| IBIS file generated by GenIBIS.exe Version 2.20
|   am37xxcbp
[IBIS ver]   4.1
[File name]   sprm509.ibs
[File Rev]   1.0
[Date]   Fri June 4, 2010, 5:00:0
[Source]   Data created at Texas Instruments
[Notes]   1) IBIS spec conformance checker (IBISCK4) ran with 0 errors
   and 576 warnings.  Warnings should be waived.
[Disclaimer] Please be aware that in the absence of a written agreement,
   Texas Instruments (TI) assumes no liability for: 1) the
   accuracy of the IBIS models provided to your company, 2) the
   proper functioning of these IBIS models in your design or for
   any resulting applications, or, 3) infringement of patents,
   copyrights, or intellectual property rights resulting from
   your use of these IBIS models. TI provides IBIS models as a
   service to our customers and therefore reserves the right to
   limit distribution of the IBIS models.
[Copyright]   Property of Texas Instruments Incorporated. Unauthorised
   reproduction and/or distribution is strictly prohibited. This
   product is protected under copyright law and trade secret law
   as an unpublished work. Created 1999,(C) Copyright 1999-2001,
   Texas Instruments Incorporated., All Rights Reserved. These
   commodities are under the U.S. Government distribution license
   control.As such,they are not to be re-exported without the
   prior approval of the U.S. Department of Commerce.
|   Component am37xxcbp
[Component]   am37xxcbp
[Manufacturer]   Texas Instruments.
[Package Model] am37xxcbp
[Package]
|   typ   min   max
R_pkg   0.39276334   6.43680e-004   7.84883e-001
L_pkg   4.201879E-009   -9.18420e-011   8.49560e-009
C_pkg   6.560845E-011   -1.66561e-011   1.47873e-010
[Pin]   signal_name   model_name
C27   CAM_PCLK   Selector2
C24   CAM_D3   Selector16
C23   CAM_FLD   Selector10
AH17   CAM_D1   Selector3
B26   CAM_XCLKB   Selector2
B25   CAM_D10   Selector8
A25   CAM_D5   Selector16
A24   CAM_HS   Selector10
K27   CAM_D8   Selector12
C26   CAM_D11   Selector8
D24   CAM_D4   Selector16
K28   CAM_D6   Selector12
L27   CAM_D9   Selector12
B24   CAM_D2   Selector16
L28   CAM_D7   Selector12
AG17   CAM_D0   Selector3
B23   CAM_WEN   Selector10
A23   CAM_VS   Selector10
C25   CAM_XCLKA   Selector2
D25   CAM_STROBE   Selector2
AG19   gpio_112   Selector12
AH19   gpio_113   Selector12
AG18   gpio_114   Selector12
AH18   gpio_115   Selector12
AD27   DSS_DATA11   Selector16
E27   DSS_ACBIAS   Selector8
D27   DSS_VSYNC   Selector8
H25   DSS_DATA19   Selector8
E28   DSS_DATA20   Selector8
AH23   DSS_DATA3   Selector15
H27   DSS_DATA17   Selector8
AB27   DSS_DATA13   Selector16
AC27   DSS_DATA22   Selector16
AG23   DSS_DATA2   Selector15
AD28   DSS_DATA10   Selector16
G26   DSS_DATA9   Selector8
AA27   DSS_DATA15   Selector16
AH24   DSS_DATA5   Selector15
D26   DSS_HSYNC   Selector8
AG22   DSS_DATA0   Selector13
AG24   DSS_DATA4   Selector15
H26   DSS_DATA18   Selector8
AB28   DSS_DATA12   Selector16
AH22   DSS_DATA1   Selector13
F28   DSS_DATA7   Selector8
AA28   DSS_DATA14   Selector16
G25   DSS_DATA16   Selector8
D28   DSS_PCLK   Selector8
J26   DSS_DATA21   Selector8
E26   DSS_DATA6   Selector8
AC28   DSS_DATA23   Selector16
F27   DSS_DATA8   Selector8
AE10   ETK_CTL   Selector2
AH12   ETK_D2   Selector2
AG7   ETK_D12   Selector2
AG8   ETK_D14   Selector2
AE11   ETK_D4   Selector2
AH8   ETK_D15   Selector2
AE7   ETK_D10   Selector2
AH7   ETK_D13   Selector2
AF11   ETK_D0   Selector2
AF10   ETK_CLK   Selector2
AG9   ETK_D9   Selector2
AG12   ETK_D1   Selector2
AE13   ETK_D3   Selector2
AH14   ETK_D7   Selector2
AF9   ETK_D8   Selector2
AF7   ETK_D11   Selector2
AH9   ETK_D5   Selector2
AF13   ETK_D6   Selector2
K8   GPMC_WAIT2   Selector16
T2   GPMC_D13   Selector8
U8   GPMC_NCS3   Selector16
M3   GPMC_A8   Selector16
V2   GPMC_D6   Selector8
H2   GPMC_D8   Selector8
L4   GPMC_A3   Selector8
H1   GPMC_NWP   Selector8
R8   GPMC_NCS5   Selector16
G3   GPMC_NBE0_CLE   Selector8
L3   GPMC_A9   Selector16
P8   GPMC_NCS6   Selector16
R3   GPMC_A6   Selector16
Y1   GPMC_D15   Selector8
H3   GPMC_NCS1   Selector16
T1   GPMC_D4   Selector8
K3   GPMC_A10   Selector16
L8   GPMC_WAIT1   Selector16
K1   GPMC_D0   Selector8
F3   GPMC_NADV_ALE   Selector16
V1   GPMC_D5   Selector8
R1   GPMC_D11   Selector8
T8   GPMC_NCS4   Selector16
L1   GPMC_D1   Selector8
G2   GPMC_NOE   Selector16
W2   GPMC_D7   Selector8
J8   GPMC_WAIT3   Selector16
M4   GPMC_A2   Selector8
P2   GPMC_D3   Selector8
K2   GPMC_D9   Selector8
W1   GPMC_D14   Selector8
K4   GPMC_A4   Selector8
G4   GPMC_NCS0   Selector16
M8   GPMC_WAIT0   Selector16
N3   GPMC_A7   Selector16
R2   GPMC_D12   Selector8
F4   GPMC_NWE   Selector16
U3   GPMC_NBE1   Selector8
N4   GPMC_A1   Selector8
V8   GPMC_NCS2   Selector16
T4   GPMC_CLK   Selector8
L2   GPMC_D2   Selector8
N8   GPMC_NCS7   Selector16
P1   GPMC_D10   Selector8
T3   GPMC_A5   Selector8
J25   HDQ_SIO   Selector5
U26   HSUSB0_DATA3   Selector2
R28   HSUSB0_DIR   Selector2
T27   HSUSB0_DATA0   Selector2
U27   HSUSB0_DATA2   Selector2
V28   HSUSB0_DATA5   Selector2
T25   HSUSB0_STP   Selector2
T26   HSUSB0_NXT   Selector2
U28   HSUSB0_DATA1   Selector2
U25   HSUSB0_DATA4   Selector2
V26   HSUSB0_DATA7   Selector2
T28   HSUSB0_CLK   Selector19
V27   HSUSB0_DATA6   Selector2
AF15   I2C2_SCL   Selector17
AG14   I2C3_SDA   Selector17
AD26   I2C4_SCL   Selector20
AF14   I2C3_SCL   Selector17
AE26   I2C4_SDA   Selector20
J21   I2C1_SDA   Selector17
AE15   I2C2_SDA   Selector17
K21   I2C1_SCL   Selector17
AA20   JTAG_TDI   Selector1
AA11   JTAG_EMU0   Selector1
AA12   JTAG_RTCK   Selector1
AA19   JTAG_TDO   Selector1
AA10   JTAG_EMU1   Selector1
AA13   JTAG_TCK   Selector1
AA18   JTAG_TMS_TMSC   Selector1
AA17   JTAG_NTRST   Selector1
T21   MCBSP_CLKS   Selector2
K26   MCBSP1_FSX   Selector2
W21   MCBSP1_CLKX   Selector2
AA21   MCBSP1_FSR   Selector2
V21   MCBSP1_DX   Selector2
Y21   MCBSP1_CLKR   Selector2
U21   MCBSP1_DR   Selector2
N21   MCBSP2_CLKX   Selector2
P21   MCBSP2_FSX   Selector2
R21   MCBSP2_DR   Selector2
M21   MCBSP2_DX   Selector2
AE5   MCBSP3_FSX   Selector2
AF5   MCBSP3_CLKX   Selector2
AF6   MCBSP3_DX   Selector2
AE6   MCBSP3_DR   Selector2
AD1   MCBSP4_DR   Selector2
AE1   MCBSP4_CLKX   Selector2
AD2   MCBSP4_DX   Selector2
AC1   MCBSP4_FSX   Selector2
AB1   MCSPI1_CS2   Selector2
AB2   MCSPI1_CS3   Selector2
AB4   MCSPI1_SIMO   Selector2
AC3   MCSPI1_CS1   Selector2
AA4   MCSPI1_SOMI   Selector2
AB3   MCSPI1_CLK   Selector2
AC2   MCSPI1_CS0   Selector2
AA3   MCSPI2_CLK   Selector2
V3   MCSPI2_CS1   Selector2
Y4   MCSPI2_CS0   Selector2
Y3   MCSPI2_SOMI   Selector2
Y2   MCSPI2_SIMO   Selector2
M27   MMC1_CMD   Selector14
N25   MMC1_DAT2   Selector14
N28   MMC1_CLK   Selector14
N27   MMC1_DAT0   Selector14
N26   MMC1_DAT1   Selector14
P28   MMC1_DAT3   Selector14
AE4   MMC2_DAT4   Selector2
AH4   MMC2_DAT1   Selector2
AG5   MMC2_CMD   Selector2
AH5   MMC2_DAT0   Selector2
AF3   MMC2_DAT6   Selector2
AF4   MMC2_DAT3   Selector2
AE2   MMC2_CLK   Selector2
AG4   MMC2_DAT2   Selector2
AE3   MMC2_DAT7   Selector2
AH3   MMC2_DAT5   Selector2
R27   gpio_128   Selector4
R25   gpio_129   Selector6
P27   gpio_126   Selector6
P26   gpio_127   Selector6
AF25   SYS_CLKREQ   Selector7
AG26   SYS_BOOT1   Selector8
AF18   SYS_BOOT3   Selector8
AH25   SYS_NRESPWRON   Model225
AE25   SYS_32K   Selector7
AF26   SYS_NIRQ   Selector18
AE21   SYS_BOOT5   Selector8
AF24   SYS_NRESWARM   Selector9
AE17   SYS_XTALIN   Model1
AG25   SYS_CLKOUT1   Selector11
AE14   SYS_BOOT2   Selector8
AF21   SYS_BOOT6   Selector16
AF19   SYS_BOOT4   Selector8
AH26   SYS_BOOT0   Selector8
AF22   SYS_OFF_MODE   Selector11
AE22   SYS_CLKOUT2   Selector10
Y8   UART1_RTS   Selector2
AA9   UART1_RX   Selector2
AA8   UART1_TX   Selector2
W8   UART1_CTS   Selector2
AB25   UART2_RTS   Selector10
AB26   UART2_CTS   Selector10
AA25   UART2_TX   Selector10
AD25   UART2_RX   Selector10
H20   UART3_RX_IRRX   Selector5
H21   UART3_TX_IRTX   Selector21
H18   UART3_CTS_RCTX   Selector5
H19   UART3_RTS_SD   Selector21
| Device pads which are not required to be modeled. Included for completeness
|U4   CAP_VDD_BB_MPU_IVA   POWER
|AH20   CAP_VDDU_ARRAY   POWER
|L21   CAP_VDD_SRAM_CORE   POWER
|AA15   CAP_VDDU_WKUP_LOGIC  POWER
|V4   CAP_VDD_SRAM_MPU_IVA POWER
|Y17   SYS_XTALGND   KELVINGROUND
|AC4   VDD_CORE   POWER
|AE18   VDD_CORE   POWER
|AE19   VDD_CORE   POWER
|AE24   VDD_CORE   POWER
|AE9   VDD_CORE   POWER
|D15   VDD_CORE   POWER
|D22   VDD_CORE   POWER
|D23   VDD_CORE   POWER
|D8   VDD_CORE   POWER
|D9   VDD_CORE   POWER
|E25   VDD_CORE   POWER
|H4   VDD_CORE   POWER
|J18   VDD_CORE   POWER
|J19   VDD_CORE   POWER
|J20   VDD_CORE   POWER
|J4   VDD_CORE   POWER
|K18   VDD_CORE   POWER
|K20   VDD_CORE   POWER
|L25   VDD_CORE   POWER
|M19   VDD_CORE   POWER
|M25   VDD_CORE   POWER
|N19   VDD_CORE   POWER
|N20   VDD_CORE   POWER
|P20   VDD_CORE   POWER
|T19   VDD_CORE   POWER
|U19   VDD_CORE   POWER
|U20   VDD_CORE   POWER
|V20   VDD_CORE   POWER
|W18   VDD_CORE   POWER
|W20   VDD_CORE   POWER
|Y16   VDD_CORE   POWER
|Y18   VDD_CORE   POWER
|Y19   VDD_CORE   POWER
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[Model Selector] Selector1
Model2 1.8V-I/O-PD-X-1.8V +5/-10%
Model3 1.8V-I/O-PI-X-1.8V +5/-10%V
Model4 1.8V-I/O-PU-X-1.8V +5/-10%
|   Usage I#1.8V#PD/PI/PU#LB0/LB1#BQ1850OMAPSMART2HYFBPB_SSBHH
[Model Selector] Selector2
Model10 1.8V-I/O-PI-LB1-1.8 +5/-10%
Model5 1.8V-I/O-PI-LB0-1.8 +5/-10%
Model6 1.8V-I/O-PU-LB0-1.8 +5/-10%
Model7 1.8V-I/O-PD-LB0-1.8 +5/-10%
Model8 1.8V-I/O-PU-LB1-1.8 +5/-10%
Model9 1.8V-I/O-PD-LB1-1.8 +5/-10%
|   Usage I#1.8V#PD/PI/PU##CAMERARX_ADDON.DY3
[Model Selector] Selector3
Model11 1.8V-INPUT-PD-X-1.8V +5/-10%
Model12 1.8V-INPUT-PI-X-1.8V +5/-10%
Model13 1.8V-INPUT-PU-X-1.8V +5/-10%
|   Usage O#1.8V#PD/PI/PU#SC00LB00/SC00LB01/SC01LB10/SC01LB11/SC10LB10/SC10LB11#BQ18OMAPSMART1HYFBPBNOPM_SSBHH
[Model Selector] Selector4
Model14 1.8V-I/O-PI-SC00LB00-1.8 +5/-10%
Model15 1.8V-I/O-PU-SC00LB00-1.8 +5/-10%
Model16 1.8V-I/O-PD-SC00LB00-1.8 +5/-10%
Model17 1.8V-I/O-PU-SC00LB01-1.8 +5/-10%
Model18 1.8V-I/O-PD-SC00LB01-1.8 +5/-10%
Model19 1.8V-I/O-PI-SC00LB01-1.8 +5/-10%
Model20 1.8V-I/O-PD-SC01LB10-1.8 +5/-10%
Model21 1.8V-I/O-PI-SC01LB10-1.8 +5/-10%
Model22 1.8V-I/O-PU-SC01LB10-1.8 +5/-10%
Model23 1.8V-I/O-PD-SC01LB11-1.8 +5/-10%
Model24 1.8V-I/O-PU-SC01LB11-1.8 +5/-10%
Model25 1.8V-I/O-PI-SC01LB11-1.8 +5/-10%
Model26 1.8V-I/O-PI-SC10LB10-1.8 +5/-10%
Model27 1.8V-I/O-PU-SC10LB10-1.8 +5/-10%
Model28 1.8V-I/O-PD-SC10LB10-1.8 +5/-10%
Model29 1.8V-I/O-PU-SC10LB11-1.8 +5/-10%
Model30 1.8V-I/O-PI-SC10LB11-1.8 +5/-10%
Model31 1.8V-I/O-PD-SC10LB11-1.8 +5/-10%
|   Usage I#1.8V#PD/PI/PU#SC00LB00/SC00LB01/SC01LB10/SC01LB11/SC10LB10/SC10LB11#BQ18OMAPSMART1HYFBPB_SSBHH
[Model Selector] Selector5
Model32 1.8V-I/O-PD-SC01LB11-1.8 +5/-10%
Model33 1.8V-I/O-PD-SC01LB10-1.8 +5/-10%
Model34 1.8V-I/O-PD-SC00LB11-1.8 +5/-10%
Model35 1.8V-I/O-PD-SC00LB10-1.8 +5/-10%
Model36 1.8V-I/O-PD-SC00LB01-1.8 +5/-10%
Model37 1.8V-I/O-PD-SC10LB01-1.8 +5/-10%
Model38 1.8V-I/O-PD-SC10LB00-1.8 +5/-10%
Model39 1.8V-I/O-PD-SC01LB01-1.8 +5/-10%
Model40 1.8V-I/O-PD-SC01LB00-1.8 +5/-10%
Model41 1.8V-I/O-PD-SC00LB00-1.8 +5/-10%
Model42 1.8V-I/O-PD-SC10LB11-1.8 +5/-10%
Model43 1.8V-I/O-PD-SC10LB10-1.8 +5/-10%
Model44 1.8V-I/O-PI-SC10LB10-1.8 +5/-10%
Model45 1.8V-I/O-PI-SC10LB01-1.8 +5/-10%
Model46 1.8V-I/O-PI-SC10LB00-1.8 +5/-10%
Model47 1.8V-I/O-PI-SC01LB10-1.8 +5/-10%
Model48 1.8V-I/O-PI-SC01LB01-1.8 +5/-10%
Model49 1.8V-I/O-PI-SC01LB00-1.8 +5/-10%
Model50 1.8V-I/O-PI-SC00LB01-1.8 +5/-10%
Model51 1.8V-I/O-PI-SC00LB00-1.8 +5/-10%
Model52 1.8V-I/O-PI-SC10LB11-1.8 +5/-10%
Model53 1.8V-I/O-PI-SC01LB11-1.8 +5/-10%
Model54 1.8V-I/O-PI-SC00LB11-1.8 +5/-10%
Model55 1.8V-I/O-PI-SC00LB10-1.8 +5/-10%
Model56 1.8V-I/O-PU-SC00LB01-1.8 +5/-10%
Model57 1.8V-I/O-PU-SC10LB11-1.8 +5/-10%
Model58 1.8V-I/O-PU-SC10LB10-1.8 +5/-10%
Model59 1.8V-I/O-PU-SC01LB11-1.8 +5/-10%
Model60 1.8V-I/O-PU-SC01LB10-1.8 +5/-10%
Model61 1.8V-I/O-PU-SC00LB00-1.8 +5/-10%
Model62 1.8V-I/O-PU-SC10LB01-1.8 +5/-10%
Model63 1.8V-I/O-PU-SC10LB00-1.8 +5/-10%
Model64 1.8V-I/O-PU-SC00LB11-1.8 +5/-10%
Model65 1.8V-I/O-PU-SC01LB01-1.8 +5/-10%
Model66 1.8V-I/O-PU-SC00LB10-1.8 +5/-10%
Model67 1.8V-I/O-PU-SC01LB00-1.8 +5/-10%
|   Usage IO#1.8V/3V#PD/PI/PU##BQUSIM1833DVHYPBFZLP18NOPM_SSCHH
[Model Selector] Selector6
Model68 1.8V-I/O-PD-X-+5/-10%V
Model69 1.8V-I/O-PU-X-+5/-10%V
Model70 1.8V-I/O-PI-X-+5/-10%V
Model71 3V-I/O-PD-X-3V+-10%
Model72 3V-I/O-PU-X-3V+-10%
Model73 3V-I/O-PI-X-3V+-10%
|   Usage I#1.8V#PD/PI/PU#SC00LB00/SC00LB01/SC01LB10/SC01LB11/SC10LB10/SC10LB11#BQ18OMAPSMART1HYFBPBNOPM_SSBHV
[Model Selector] Selector7
Model100 1.8V-I/O-PU-SC10LB10-1.8 +5/-10%
Model101 1.8V-I/O-PU-SC01LB11-1.8 +5/-10%
Model102 1.8V-I/O-PU-SC01LB10-1.8 +5/-10%
Model103 1.8V-I/O-PU-SC00LB00-1.8 +5/-10%
Model104 1.8V-I/O-PU-SC10LB01-1.8 +5/-10%
Model105 1.8V-I/O-PU-SC10LB00-1.8 +5/-10%
Model106 1.8V-I/O-PU-SC00LB11-1.8 +5/-10%
Model107 1.8V-I/O-PU-SC01LB01-1.8 +5/-10%
Model108 1.8V-I/O-PU-SC00LB10-1.8 +5/-10%
Model109 1.8V-I/O-PU-SC01LB00-1.8 +5/-10%
Model74 1.8V-I/O-PD-SC01LB11-1.8 +5/-10%
Model75 1.8V-I/O-PD-SC01LB10-1.8 +5/-10%
Model76 1.8V-I/O-PD-SC00LB11-1.8 +5/-10%
Model77 1.8V-I/O-PD-SC00LB10-1.8 +5/-10%
Model78 1.8V-I/O-PD-SC00LB01-1.8 +5/-10%
Model79 1.8V-I/O-PD-SC10LB01-1.8 +5/-10%
Model80 1.8V-I/O-PD-SC10LB00-1.8 +5/-10%
Model81 1.8V-I/O-PD-SC01LB01-1.8 +5/-10%
Model82 1.8V-I/O-PD-SC01LB00-1.8 +5/-10%
Model83 1.8V-I/O-PD-SC00LB00-1.8 +5/-10%
Model84 1.8V-I/O-PD-SC10LB11-1.8 +5/-10%
Model85 1.8V-I/O-PD-SC10LB10-1.8 +5/-10%
Model86 1.8V-I/O-PI-SC10LB10-1.8 +5/-10%
Model87 1.8V-I/O-PI-SC10LB01-1.8 +5/-10%
Model88 1.8V-I/O-PI-SC10LB00-1.8 +5/-10%
Model89 1.8V-I/O-PI-SC01LB10-1.8 +5/-10%
Model90 1.8V-I/O-PI-SC01LB01-1.8 +5/-10%
Model91 1.8V-I/O-PI-SC01LB00-1.8 +5/-10%
Model92 1.8V-I/O-PI-SC00LB01-1.8 +5/-10%
Model93 1.8V-I/O-PI-SC00LB00-1.8 +5/-10%
Model94 1.8V-I/O-PI-SC10LB11-1.8 +5/-10%
Model95 1.8V-I/O-PI-SC01LB11-1.8 +5/-10%
Model96 1.8V-I/O-PI-SC00LB11-1.8 +5/-10%
Model97 1.8V-I/O-PI-SC00LB10-1.8 +5/-10%
Model98 1.8V-I/O-PU-SC00LB01-1.8 +5/-10%
Model99 1.8V-I/O-PU-SC10LB11-1.8 +5/-10%
|   Usage O#1.8V#PD/PI/PU#LB0/LB1#BQ18OMAPSMART2HYFBPB_SSBHH
[Model Selector] Selector8
Model110 1.8V-I/O-PD-LB1-1.8 +5/-10%
Model111 1.8V-I/O-PD-LB0-1.8 +5/-10%
Model112 1.8V-I/O-PI-LB0-1.8 +5/-10%
Model113 1.8V-I/O-PI-LB1-1.8 +5/-10%
Model114 1.8V-I/O-PU-LB1-1.8 +5/-10%
Model115 1.8V-I/O-PU-LB0-1.8 +5/-10%
|   Usage IO#1.8V#PD/PI/PU##BQOMAPGFR50CHYFBPBNOPM_SSBHV
[Model Selector] Selector9
Model116 1.8V-I/O-PD-X-+5/-10%V
Model117 1.8V-I/O-PI-X-+5/-10%V
Model118 1.8V-I/O-PU-X-+5/-10%V
|   Usage IO#1.8V#PD/PI/PU#LB0/LB1#BQ1850OMAPSMART2HYFBPB_SSBHV
[Model Selector] Selector10
Model119 1.8V-I/O-PI-LB0-1.8 +5/-10%
Model120 1.8V-I/O-PU-LB0-1.8 +5/-10%
Model121 1.8V-I/O-PD-LB0-1.8 +5/-10%
Model122 1.8V-I/O-PU-LB1-1.8 +5/-10%
Model123 1.8V-I/O-PD-LB1-1.8 +5/-10%
Model124 1.8V-I/O-PI-LB1-1.8 +5/-10%
|   Usage O#1.8V#PD/PI/PU#SC00LB00/SC00LB01/SC01LB10/SC01LB11/SC10LB10/SC10LB11#BQ18OMAPSMART1HYFBPBNOPM_SSBHV
[Model Selector] Selector11
Model100 1.8V-I/O-PU-SC10LB10-1.8 +5/-10%
Model101 1.8V-I/O-PU-SC01LB11-1.8 +5/-10%
Model102 1.8V-I/O-PU-SC01LB10-1.8 +5/-10%
Model103 1.8V-I/O-PU-SC00LB00-1.8 +5/-10%
Model74 1.8V-I/O-PD-SC01LB11-1.8 +5/-10%
Model75 1.8V-I/O-PD-SC01LB10-1.8 +5/-10%
Model78 1.8V-I/O-PD-SC00LB01-1.8 +5/-10%
Model83 1.8V-I/O-PD-SC00LB00-1.8 +5/-10%
Model84 1.8V-I/O-PD-SC10LB11-1.8 +5/-10%
Model85 1.8V-I/O-PD-SC10LB10-1.8 +5/-10%
Model86 1.8V-I/O-PI-SC10LB10-1.8 +5/-10%
Model89 1.8V-I/O-PI-SC01LB10-1.8 +5/-10%
Model92 1.8V-I/O-PI-SC00LB01-1.8 +5/-10%
Model93 1.8V-I/O-PI-SC00LB00-1.8 +5/-10%
Model94 1.8V-I/O-PI-SC10LB11-1.8 +5/-10%
Model95 1.8V-I/O-PI-SC01LB11-1.8 +5/-10%
Model98 1.8V-I/O-PU-SC00LB01-1.8 +5/-10%
Model99 1.8V-I/O-PU-SC10LB11-1.8 +5/-10%
|   Usage I#1.8V#PD/PI/PU##CAMERARX_CORE.YAGPI
[Model Selector] Selector12
Model125 1.8V-INPUT-PD-X-1.8V +5/-10%
Model126 1.8V-INPUT-PI-X-1.8V +5/-10%
Model127 1.8V-INPUT-PU-X-1.8V +5/-10%
|   Usage IO#1.8V#PD/PI/PU#SC00LB00/SC00LB01/SC01LB10/SC01LB11/SC10LB10/SC10LB11#DSIPHY_WIO_ADDON_GPIOWRAPPER.GPI
[Model Selector] Selector13
Model128 1.8V-I/O-PD-SC01LB11-1.8 +5/-10%
Model129 1.8V-I/O-PD-SC01LB10-1.8 +5/-10%
Model130 1.8V-I/O-PD-SC00LB11-1.8 +5/-10%
Model131 1.8V-I/O-PD-SC00LB10-1.8 +5/-10%
Model132 1.8V-I/O-PD-SC00LB01-1.8 +5/-10%
Model133 1.8V-I/O-PD-SC10LB01-1.8 +5/-10%
Model134 1.8V-I/O-PD-SC10LB00-1.8 +5/-10%
Model135 1.8V-I/O-PD-SC01LB01-1.8 +5/-10%
Model136 1.8V-I/O-PD-SC01LB00-1.8 +5/-10%
Model137 1.8V-I/O-PD-SC00LB00-1.8 +5/-10%
Model138 1.8V-I/O-PD-SC10LB11-1.8 +5/-10%
Model139 1.8V-I/O-PD-SC10LB10-1.8 +5/-10%
Model140 1.8V-I/O-PI-SC10LB10-1.8 +5/-10%
Model141 1.8V-I/O-PI-SC10LB01-1.8 +5/-10%
Model142 1.8V-I/O-PI-SC10LB00-1.8 +5/-10%
Model143 1.8V-I/O-PI-SC01LB10-1.8 +5/-10%
Model144 1.8V-I/O-PI-SC01LB01-1.8 +5/-10%
Model145 1.8V-I/O-PI-SC01LB00-1.8 +5/-10%
Model146 1.8V-I/O-PI-SC00LB01-1.8 +5/-10%
Model147 1.8V-I/O-PI-SC00LB00-1.8 +5/-10%
Model148 1.8V-I/O-PI-SC10LB11-1.8 +5/-10%
Model149 1.8V-I/O-PI-SC01LB11-1.8 +5/-10%
Model150 1.8V-I/O-PI-SC00LB11-1.8 +5/-10%
Model151 1.8V-I/O-PI-SC00LB10-1.8 +5/-10%
Model152 1.8V-I/O-PU-SC00LB01-1.8 +5/-10%
Model153 1.8V-I/O-PU-SC10LB11-1.8 +5/-10%
Model154 1.8V-I/O-PU-SC10LB10-1.8 +5/-10%
Model155 1.8V-I/O-PU-SC01LB11-1.8 +5/-10%
Model156 1.8V-I/O-PU-SC01LB10-1.8 +5/-10%
Model157 1.8V-I/O-PU-SC00LB00-1.8 +5/-10%
Model158 1.8V-I/O-PU-SC10LB01-1.8 +5/-10%
Model159 1.8V-I/O-PU-SC10LB00-1.8 +5/-10%
Model160 1.8V-I/O-PU-SC00LB11-1.8 +5/-10%
Model161 1.8V-I/O-PU-SC01LB01-1.8 +5/-10%
Model162 1.8V-I/O-PU-SC00LB10-1.8 +5/-10%
Model163 1.8V-I/O-PU-SC01LB00-1.8 +5/-10%
|   Usage O#1.8V/3V#PD/PI/PU#SC0/SC1#BQMMC1833DVHYPBFZLP18_SSCHH
[Model Selector] Selector14
Model200 1.8V-I/O-PD-SC0-1.8V +5/-10%
Model201 1.8V-I/O-PD-SC1-1.8V +5/-10%
Model202 1.8V-I/O-PI-SC0-1.8V +5/-10%
Model203 1.8V-I/O-PI-SC1-1.8V +5/-10%
Model204 1.8V-I/O-PU-SC0-1.8V +5/-10%
Model205 1.8V-I/O-PU-SC1-1.8V +5/-10%
Model206 3V-I/O-PD-SC0-3V +-10%
Model207 3V-I/O-PD-SC1-3V +-10%
Model208 3V-I/O-PI-SC0-3V +-10%
Model209 3V-I/O-PI-SC1-3V +-10%
Model210 3V-I/O-PU-SC0-3V +-10%
Model211 3V-I/O-PU-SC1-3V +-10%
|   Usage IO#1.8V#PD/PI/PU#SC00LB00/SC00LB01/SC01LB10/SC01LB11/SC10LB10/SC10LB11#DSIPHY_WIO_CORE_GPIOWRAPPER.GPI
[Model Selector] Selector15
Model164 1.8V-I/O-PD-SC01LB11-1.8 +5/-10%
Model165 1.8V-I/O-PD-SC01LB10-1.8 +5/-10%
Model166 1.8V-I/O-PD-SC00LB11-1.8 +5/-10%
Model167 1.8V-I/O-PD-SC00LB10-1.8 +5/-10%
Model168 1.8V-I/O-PD-SC00LB01-1.8 +5/-10%
Model169 1.8V-I/O-PD-SC10LB01-1.8 +5/-10%
Model170 1.8V-I/O-PD-SC10LB00-1.8 +5/-10%
Model171 1.8V-I/O-PD-SC01LB01-1.8 +5/-10%
Model172 1.8V-I/O-PD-SC01LB00-1.8 +5/-10%
Model173 1.8V-I/O-PD-SC00LB00-1.8 +5/-10%
Model174 1.8V-I/O-PD-SC10LB11-1.8 +5/-10%
Model175 1.8V-I/O-PD-SC10LB10-1.8 +5/-10%
Model176 1.8V-I/O-PI-SC10LB10-1.8 +5/-10%
Model177 1.8V-I/O-PI-SC10LB01-1.8 +5/-10%
Model178 1.8V-I/O-PI-SC10LB00-1.8 +5/-10%
Model179 1.8V-I/O-PI-SC01LB10-1.8 +5/-10%
Model180 1.8V-I/O-PI-SC01LB01-1.8 +5/-10%
Model181 1.8V-I/O-PI-SC01LB00-1.8 +5/-10%
Model182 1.8V-I/O-PI-SC00LB01-1.8 +5/-10%
Model183 1.8V-I/O-PI-SC00LB00-1.8 +5/-10%
Model184 1.8V-I/O-PI-SC10LB11-1.8 +5/-10%
Model185 1.8V-I/O-PI-SC01LB11-1.8 +5/-10%
Model186 1.8V-I/O-PI-SC00LB11-1.8 +5/-10%
Model187 1.8V-I/O-PI-SC00LB10-1.8 +5/-10%
Model188 1.8V-I/O-PU-SC00LB01-1.8 +5/-10%
Model189 1.8V-I/O-PU-SC10LB11-1.8 +5/-10%
Model190 1.8V-I/O-PU-SC10LB10-1.8 +5/-10%
Model191 1.8V-I/O-PU-SC01LB11-1.8 +5/-10%
Model192 1.8V-I/O-PU-SC01LB10-1.8 +5/-10%
Model193 1.8V-I/O-PU-SC00LB00-1.8 +5/-10%
Model194 1.8V-I/O-PU-SC10LB01-1.8 +5/-10%
Model195 1.8V-I/O-PU-SC10LB00-1.8 +5/-10%
Model196 1.8V-I/O-PU-SC00LB11-1.8 +5/-10%
Model197 1.8V-I/O-PU-SC01LB01-1.8 +5/-10%
Model198 1.8V-I/O-PU-SC00LB10-1.8 +5/-10%
Model199 1.8V-I/O-PU-SC01LB00-1.8 +5/-10%
|   Usage I#1.8V#PD/PI/PU#LB0/LB1#BQ18OMAPSMART2HYFBPB_SSBHV
[Model Selector] Selector16
Model212 1.8V-I/O-PD-LB1-1.8 +5/-10%
Model213 1.8V-I/O-PD-LB0-1.8 +5/-10%
Model214 1.8V-I/O-PI-LB0-1.8 +5/-10%
Model215 1.8V-I/O-PI-LB1-1.8 +5/-10%
Model216 1.8V-I/O-PU-LB1-1.8 +5/-10%
Model217 1.8V-I/O-PU-LB0-1.8 +5/-10%
|   Usage IO#1.8V#PI/PU#LB00/LB01/LB10#BQOMAPI2CHYFBPBRES_SSBHH
[Model Selector] Selector17
Model218 1.8V-I/O_OPEN_DRAIN-PI-LB00-1.8V +5/-10%
Model219 1.8V-I/O_OPEN_DRAIN-PI-LB00-1.8V +5/-10%
Model220 1.8V-I/O-PU-LB00-1.8V +5/-10%
Model221 1.8V-I/O_OPEN_DRAIN-PU-LB01-1.8V +5/-10%
Model222 1.8V-I/O_OPEN_DRAIN-PU-LB10-1.8V +5/-10%
Model223 1.8V-I/O_OPEN_DRAIN-PU-LB00-1.8V +5/-10%
Model224 1.8V-I/O_OPEN_DRAIN-PU-LB00-1.8V +5/-10%
|   Usage I#1.8V#PD/PI/PU#SC00LB00/SC00LB01/SC01LB10/SC01LB11/SC10LB10/SC10LB11#BQ18OMAPSMART1HYFBPB_SSBHV
[Model Selector] Selector18
Model232 1.8V-I/O-PD-SC01LB11-1.8 +5/-10%
Model233 1.8V-I/O-PD-SC01LB10-1.8 +5/-10%
Model234 1.8V-I/O-PD-SC00LB11-1.8 +5/-10%
Model235 1.8V-I/O-PD-SC00LB01-1.8 +5/-10%
Model236 1.8V-I/O-PD-SC10LB01-1.8 +5/-10%
Model237 1.8V-I/O-PD-SC10LB00-1.8 +5/-10%
Model238 1.8V-I/O-PD-SC01LB01-1.8 +5/-10%
Model239 1.8V-I/O-PD-SC00LB00-1.8 +5/-10%
Model240 1.8V-I/O-PD-SC10LB11-1.8 +5/-10%
Model241 1.8V-I/O-PD-SC10LB10-1.8 +5/-10%
Model242 1.8V-I/O-PI-SC10LB10-1.8 +5/-10%
Model243 1.8V-I/O-PI-SC10LB01-1.8 +5/-10%
Model244 1.8V-I/O-PI-SC10LB00-1.8 +5/-10%
Model245 1.8V-I/O-PI-SC01LB10-1.8 +5/-10%
Model246 1.8V-I/O-PI-SC01LB01-1.8 +5/-10%
Model247 1.8V-I/O-PI-SC00LB01-1.8 +5/-10%
Model248 1.8V-I/O-PI-SC00LB00-1.8 +5/-10%
Model249 1.8V-I/O-PI-SC10LB11-1.8 +5/-10%
Model250 1.8V-I/O-PI-SC01LB11-1.8 +5/-10%
Model251 1.8V-I/O-PI-SC00LB11-1.8 +5/-10%
Model252 1.8V-I/O-PI-SC00LB10-1.8 +5/-10%
Model253 1.8V-I/O-PU-SC00LB01-1.8 +5/-10%
Model254 1.8V-I/O-PU-SC10LB11-1.8 +5/-10%
Model255 1.8V-I/O-PU-SC10LB10-1.8 +5/-10%
Model256 1.8V-I/O-PU-SC01LB11-1.8 +5/-10%
Model257 1.8V-I/O-PU-SC01LB10-1.8 +5/-10%
Model258 1.8V-I/O-PU-SC00LB00-1.8 +5/-10%
Model259 1.8V-I/O-PU-SC10LB01-1.8 +5/-10%
Model260 1.8V-I/O-PU-SC10LB00-1.8 +5/-10%
Model261 1.8V-I/O-PU-SC00LB11-1.8 +5/-10%
Model262 1.8V-I/O-PU-SC01LB01-1.8 +5/-10%
Model263 1.8V-I/O-PU-SC00LB10-1.8 +5/-10%
Model264 1.8V-I/O-PU-SC01LB00-1.8 +5/-10%
|   Usage I#1.8V#PD/PI/PU#LB0/LB1#BQ18OMAPSMART2FBPB_SSBHH
[Model Selector] Selector19
Model226 1.8V-I/O-PD-LB1-1.8 +5/-10%
Model227 1.8V-I/O-PD-LB0-1.8 +5/-10%
Model228 1.8V-I/O-PI-LB0-1.8 +5/-10%
Model229 1.8V-I/O-PI-LB1-1.8 +5/-10%
Model230 1.8V-I/O-PU-LB1-1.8 +5/-10%
Model231 1.8V-I/O-PU-LB0-1.8 +5/-10%
|   Usage IO#1.8V#PI/PU#LB00/LB01/LB10#BQOMAPI2CHYFBPBRESNOPM_SSBHV
[Model Selector] Selector20
Model265 1.8V-I/O_OPEN_DRAIN-PI-LB00-1.8V +5/-10%
Model266 1.8V-I/O_OPEN_DRAIN-PI-LB00-1.8V +5/-10%
Model267 1.8V-I/O-PU-LB00-1.8V +5/-10%
Model268 1.8V-I/O_OPEN_DRAIN-PU-LB01-1.8V +5/-10%
Model269 1.8V-I/O_OPEN_DRAIN-PU-LB10-1.8V +5/-10%
Model270 1.8V-I/O_OPEN_DRAIN-PU-LB00-1.8V +5/-10%
Model271 1.8V-I/O_OPEN_DRAIN-PU-LB00-1.8V +5/-10%
|   Usage O#1.8V#PD/PI/PU#SC00LB00/SC00LB01/SC01LB10/SC01LB11/SC10LB10/SC10LB11#BQ18OMAPSMART1HYFBPB_SSBHH
[Model Selector] Selector21
Model32 1.8V-I/O-PD-SC01LB11-1.8 +5/-10%
Model33 1.8V-I/O-PD-SC01LB10-1.8 +5/-10%
Model36 1.8V-I/O-PD-SC00LB01-1.8 +5/-10%
Model41 1.8V-I/O-PD-SC00LB00-1.8 +5/-10%
Model42 1.8V-I/O-PD-SC10LB11-1.8 +5/-10%
Model43 1.8V-I/O-PD-SC10LB10-1.8 +5/-10%
Model44 1.8V-I/O-PI-SC10LB10-1.8 +5/-10%
Model47 1.8V-I/O-PI-SC01LB10-1.8 +5/-10%
Model50 1.8V-I/O-PI-SC00LB01-1.8 +5/-10%
Model51 1.8V-I/O-PI-SC00LB00-1.8 +5/-10%
Model52 1.8V-I/O-PI-SC10LB11-1.8 +5/-10%
Model53 1.8V-I/O-PI-SC01LB11-1.8 +5/-10%
Model56 1.8V-I/O-PU-SC00LB01-1.8 +5/-10%
Model57 1.8V-I/O-PU-SC10LB11-1.8 +5/-10%
Model58 1.8V-I/O-PU-SC10LB10-1.8 +5/-10%
Model59 1.8V-I/O-PU-SC01LB11-1.8 +5/-10%
Model60 1.8V-I/O-PU-SC01LB10-1.8 +5/-10%
Model61 1.8V-I/O-PU-SC00LB00-1.8 +5/-10%
| Package model definition
[Define Package Model]  am37xxcbp
[Manufacturer]   Texas Instruments.
[OEM]   Texas Instruments.
[Description]   am37xxcbp package model generated by GenIBIS.exe
[Number Of Pins]   223
[Pin Numbers]
C27   | 1 CAM_PCLK   I
C24   | 2 CAM_D3   I
C23   | 3 CAM_FLD   IO
AH17   | 4 CAM_D1   I
B26   | 5 CAM_XCLKB   O
B25   | 6 CAM_D10   I
A25   | 7 CAM_D5   I
A24   | 8 CAM_HS   IO
K27   | 9 CAM_D8   I
C26   | 10 CAM_D11   I
D24   | 11 CAM_D4   I
K28   | 12 CAM_D6   I
L27   | 13 CAM_D9   I
B24   | 14 CAM_D2   I
L28   | 15 CAM_D7   I
AG17   | 16 CAM_D0   I
B23   | 17 CAM_WEN   I
A23   | 18 CAM_VS   IO
C25   | 19 CAM_XCLKA   O
D25   | 20 CAM_STROBE   O
AG19   | 21 gpio_112   I
AH19   | 22 gpio_113   I
AG18   | 23 gpio_114   I
AH18   | 24 gpio_115   I
AD27   | 25 DSS_DATA11   IO
E27   | 26 DSS_ACBIAS   O
D27   | 27 DSS_VSYNC   O
H25   | 28 DSS_DATA19   IO
E28   | 29 DSS_DATA20   O
AH23   | 30 DSS_DATA3   IO
H27   | 31 DSS_DATA17   IO
AB27   | 32 DSS_DATA13   IO
AC27   | 33 DSS_DATA22   O
AG23   | 34 DSS_DATA2   IO
AD28   | 35 DSS_DATA10   IO
G26   | 36 DSS_DATA9   IO
AA27   | 37 DSS_DATA15   IO
AH24   | 38 DSS_DATA5   IO
D26   | 39 DSS_HSYNC   O
AG22   | 40 DSS_DATA0   IO
AG24   | 41 DSS_DATA4   IO
H26   | 42 DSS_DATA18   IO
AB28   | 43 DSS_DATA12   IO
AH22   | 44 DSS_DATA1   IO
F28   | 45 DSS_DATA7   IO
AA28   | 46 DSS_DATA14   IO
G25   | 47 DSS_DATA16   IO
D28   | 48 DSS_PCLK   O
J26   | 49 DSS_DATA21   O
E26   | 50 DSS_DATA6   IO
AC28   | 51 DSS_DATA23   O
F27   | 52 DSS_DATA8   IO
AE10   | 53 ETK_CTL   O
AH12   | 54 ETK_D2   O
AG7   | 55 ETK_D12   O
AG8   | 56 ETK_D14   O
AE11   | 57 ETK_D4   O
AH8   | 58 ETK_D15   O
AE7   | 59 ETK_D10   O
AH7   | 60 ETK_D13   O
AF11   | 61 ETK_D0   O
AF10   | 62 ETK_CLK   O
AG9   | 63 ETK_D9   O
AG12   | 64 ETK_D1   O
AE13   | 65 ETK_D3   O
AH14   | 66 ETK_D7   O
AF9   | 67 ETK_D8   O
AF7   | 68 ETK_D11   O
AH9   | 69 ETK_D5   O
AF13   | 70 ETK_D6   O
K8   | 71 GPMC_WAIT2   I
T2   | 72 GPMC_D13   IO
U8   | 73 GPMC_NCS3   O
M3   | 74 GPMC_A8   O
V2   | 75 GPMC_D6   IO
H2   | 76 GPMC_D8   IO
L4   | 77 GPMC_A3   O
H1   | 78 GPMC_NWP   O
R8   | 79 GPMC_NCS5   O
G3   | 80 GPMC_NBE0_CLE   O
L3   | 81 GPMC_A9   O
P8   | 82 GPMC_NCS6   O
R3   | 83 GPMC_A6   O
Y1   | 84 GPMC_D15   IO
H3   | 85 GPMC_NCS1   O
T1   | 86 GPMC_D4   IO
K3   | 87 GPMC_A10   O
L8   | 88 GPMC_WAIT1   I
K1   | 89 GPMC_D0   IO
F3   | 90 GPMC_NADV_ALE   O
V1   | 91 GPMC_D5   IO
R1   | 92 GPMC_D11   IO
T8   | 93 GPMC_NCS4   O
L1   | 94 GPMC_D1   IO
G2   | 95 GPMC_NOE   O
W2   | 96 GPMC_D7   IO
J8   | 97 GPMC_WAIT3   I
M4   | 98 GPMC_A2   O
P2   | 99 GPMC_D3   IO
K2   | 100 GPMC_D9   IO
W1   | 101 GPMC_D14   IO
K4   | 102 GPMC_A4   O
G4   | 103 GPMC_NCS0   O
M8   | 104 GPMC_WAIT0   I
N3   | 105 GPMC_A7   O
R2   | 106 GPMC_D12   IO
F4   | 107 GPMC_NWE   O
U3   | 108 GPMC_NBE1   O
N4   | 109 GPMC_A1   O
V8   | 110 GPMC_NCS2   O
T4   | 111 GPMC_CLK   O
L2   | 112 GPMC_D2   IO
N8   | 113 GPMC_NCS7   O
P1   | 114 GPMC_D10   IO
T3   | 115 GPMC_A5   O
J25   | 116 HDQ_SIO   IO
U26   | 117 HSUSB0_DATA3   IO
R28   | 118 HSUSB0_DIR   I
T27   | 119 HSUSB0_DATA0   IO
U27   | 120 HSUSB0_DATA2   IO
V28   | 121 HSUSB0_DATA5   IO
T25   | 122 HSUSB0_STP   O
T26   | 123 HSUSB0_NXT   I
U28   | 124 HSUSB0_DATA1   IO
U25   | 125 HSUSB0_DATA4   IO
V26   | 126 HSUSB0_DATA7   IO
T28   | 127 HSUSB0_CLK   I
V27   | 128 HSUSB0_DATA6   IO
AF15   | 129 I2C2_SCL   IO
AG14   | 130 I2C3_SDA   IO
AD26   | 131 I2C4_SCL   IO
AF14   | 132 I2C3_SCL   IO
AE26   | 133 I2C4_SDA   IO
J21   | 134 I2C1_SDA   IO
AE15   | 135 I2C2_SDA   IO
K21   | 136 I2C1_SCL   IO
AA20   | 137 JTAG_TDI   I
AA11   | 138 JTAG_EMU0   IO
AA12   | 139 JTAG_RTCK   O
AA19   | 140 JTAG_TDO   O
AA10   | 141 JTAG_EMU1   IO
AA13   | 142 JTAG_TCK   I
AA18   | 143 JTAG_TMS_TMSC   IO
AA17   | 144 JTAG_NTRST   I
T21   | 145 MCBSP_CLKS   I
K26   | 146 MCBSP1_FSX   IO
W21   | 147 MCBSP1_CLKX   IO
AA21   | 148 MCBSP1_FSR   IO
V21   | 149 MCBSP1_DX   IO
Y21   | 150 MCBSP1_CLKR   IO
U21   | 151 MCBSP1_DR   I
N21   | 152 MCBSP2_CLKX   IO
P21   | 153 MCBSP2_FSX   IO
R21   | 154 MCBSP2_DR   I
M21   | 155 MCBSP2_DX   IO
AE5   | 156 MCBSP3_FSX   IO
AF5   | 157 MCBSP3_CLKX   IO
AF6   | 158 MCBSP3_DX   IO
AE6   | 159 MCBSP3_DR   I
AD1   | 160 MCBSP4_DR   I
AE1   | 161 MCBSP4_CLKX   IO
AD2   | 162 MCBSP4_DX   IO
AC1   | 163 MCBSP4_FSX   IO
AB1   | 164 MCSPI1_CS2   O
AB2   | 165 MCSPI1_CS3   O
AB4   | 166 MCSPI1_SIMO   IO
AC3   | 167 MCSPI1_CS1   O
AA4   | 168 MCSPI1_SOMI   IO
AB3   | 169 MCSPI1_CLK   IO
AC2   | 170 MCSPI1_CS0   IO
AA3   | 171 MCSPI2_CLK   IO
V3   | 172 MCSPI2_CS1   O
Y4   | 173 MCSPI2_CS0   IO
Y3   | 174 MCSPI2_SOMI   IO
Y2   | 175 MCSPI2_SIMO   IO
M27   | 176 MMC1_CMD   IO
N25   | 177 MMC1_DAT2   IO
N28   | 178 MMC1_CLK   O
N27   | 179 MMC1_DAT0   IO
N26   | 180 MMC1_DAT1   IO
P28   | 181 MMC1_DAT3   IO
AE4   | 182 MMC2_DAT4   IO
AH4   | 183 MMC2_DAT1   IO
AG5   | 184 MMC2_CMD   IO
AH5   | 185 MMC2_DAT0   IO
AF3   | 186 MMC2_DAT6   IO
AF4   | 187 MMC2_DAT3   IO
AE2   | 188 MMC2_CLK   O
AG4   | 189 MMC2_DAT2   IO
AE3   | 190 MMC2_DAT7   IO
AH3   | 191 MMC2_DAT5   IO
R27   | 192 gpio_128   O
R25   | 193 gpio_129   O
P27   | 194 gpio_126   IO
P26   | 195 gpio_127   O
AF25   | 196 SYS_CLKREQ   IO
AG26   | 197 SYS_BOOT1   I
AF18   | 198 SYS_BOOT3   I
AH25   | 199 SYS_NRESPWRON   I
AE25   | 200 SYS_32K   I
AF26   | 201 SYS_NIRQ   I
AE21   | 202 SYS_BOOT5   I
AF24   | 203 SYS_NRESWARM   IO
AE17   | 204 SYS_XTALIN   I
AG25   | 205 SYS_CLKOUT1   O
AE14   | 206 SYS_BOOT2   I
AF21   | 207 SYS_BOOT6   I
AF19   | 208 SYS_BOOT4   I
AH26   | 209 SYS_BOOT0   I
AF22   | 210 SYS_OFF_MODE   O
AE22   | 211 SYS_CLKOUT2   O
Y8   | 212 UART1_RTS   O
AA9   | 213 UART1_RX   I
AA8   | 214 UART1_TX   O
W8   | 215 UART1_CTS   I
AB25   | 216 UART2_RTS   O
AB26   | 217 UART2_CTS   I
AA25   | 218 UART2_TX   O
AD25   | 219 UART2_RX   I
H20   | 220 UART3_RX_IRRX   I
H21   | 221 UART3_TX_IRTX   O
H18   | 222 UART3_CTS_RCTX   IO
H19   | 223 UART3_RTS_SD   O
[Model Data]
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[End Model Data]
[End Package Model]
| Models and submodels in the file (271): Model1 (Input), Model2 (I/O), Model3 (I/O), Model4 (I/O), Model5 (I/O), Model6 (I/O), Model7 (I/O), Model8 (I/O), Model9 (I/O), Model10 (I/O), Model11 (Input), Model12 (Input), Model13 (Input), Model14 (I/O), Model15 (I/O), Model16 (I/O), Model17 (I/O), Model18 (I/O), Model19 (I/O), Model20 (I/O), Model21 (I/O), Model22 (I/O), Model23 (I/O), Model24 (I/O), Model25 (I/O), Model26 (I/O), Model27 (I/O), Model28 (I/O), Model29 (I/O), Model30 (I/O), Model31 (I/O), Model32 (I/O), Model33 (I/O), Model34 (I/O), Model35 (I/O), Model36 (I/O), Model37 (I/O), Model38 (I/O), Model39 (I/O), Model40 (I/O), Model41 (I/O), Model42 (I/O), Model43 (I/O), Model44 (I/O), Model45 (I/O), Model46 (I/O), Model47 (I/O), Model48 (I/O), Model49 (I/O), Model50 (I/O), Model51 (I/O), Model52 (I/O), Model53 (I/O), Model54 (I/O), Model55 (I/O), Model56 (I/O), Model57 (I/O), Model58 (I/O), Model59 (I/O), Model60 (I/O), Model61 (I/O), Model62 (I/O), Model63 (I/O), Model64 (I/O), Model65 (I/O), Model66 (I/O), Model67 (I/O), Model68 (I/O), Model69 (I/O), Model70 (I/O), Model71 (I/O), Model72 (I/O), Model73 (I/O), Model74 (I/O), Model75 (I/O), Model76 (I/O), Model77 (I/O), Model78 (I/O), Model79 (I/O), Model80 (I/O)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
